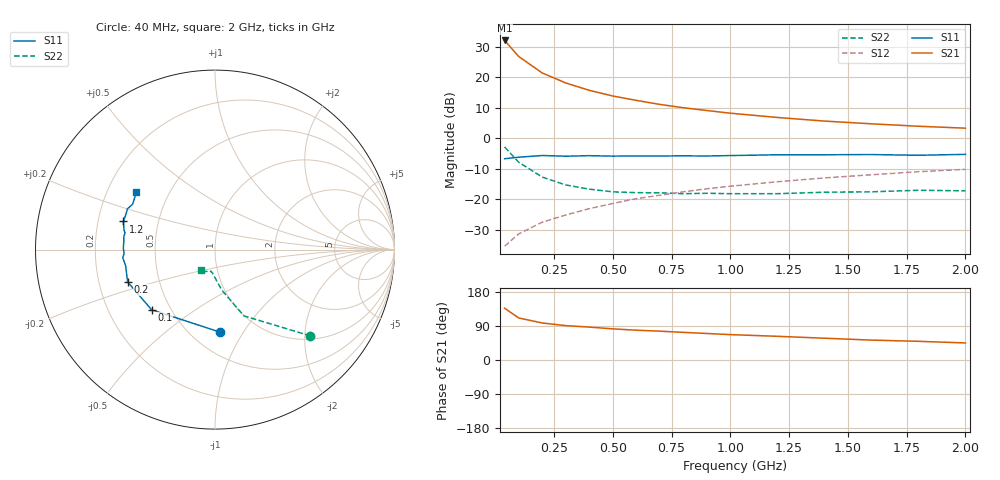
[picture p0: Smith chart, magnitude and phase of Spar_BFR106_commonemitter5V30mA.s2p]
! Filename:  BFR106B.S2P  Version:  2.0
! NXP part #: BFR106  Date: Jun 1990
! Bias condition: Vce=5V, Ic=30mA
#  MHz  S  MA  R  50
! Freq  S11  S21  S12  S22  !GUM [dB]
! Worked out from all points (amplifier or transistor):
!   16 points, 40 MHz to 2 GHz, reference 50 ohm
!   highest |S21| = 32.0 dB at 40 MHz (marker M1)
!   |S21| within 3 dB of that: start of sweep to 74.27 MHz
!   unconditionally stable (mu >= 1): 328 MHz to 1.938 GHz
!   at 200 MHz: K = 0.86, MSG = 24.4 dB, |S12| = -27.5 dB
!   at 800 MHz: K = 1.06, MAG = 12.2 dB, |S12| = -17.6 dB
!   at 2 GHz: K = 0.99, MSG = 6.7 dB, |S12| = -10.2 dB
!   S11 on the Smith chart (normalised r, x): 40 MHz: 0.68, -0.79; 100 MHz: 0.39, -0.34; 200 MHz: 0.33, -0.16; 1.2 GHz: 0.31, +0.14; 2 GHz: 0.33, +0.29
40  0.46 -86.7  39.78 136.7  0.017 63.4  0.717 -42.1
100  0.487 -136.5  21.73 110.9  0.027 56.5  0.403 -66.4
200  0.519 -159.7  11.68 97.7  0.042 63.0  0.23 -80.3
300  0.506 -169.8  8.005 90.7  0.055 66.6  0.171 -87.5
400  0.516 -175.0  6.068 86.8  0.07 69.2  0.146 -92.3
500  0.507 -177.4  4.899 82.2  0.085 70.6  0.132 -95.7
600  0.511 179.1  4.153 78.6  0.102 70.9  0.128 -97.9
700  0.51 175.4  3.568 76.1  0.116 71.1  0.127 -98.9
800  0.513 171.6  3.146 72.9  0.132 71.2  0.123 -100.1
900  0.51 169.3  2.834 70.0  0.148 71.2  0.125 -99.7
1000  0.518 168.1  2.561 67.0  0.163 70.2  0.123 -101.6
1200  0.534 162.9  2.18 62.5  0.193 69.3  0.123 -106.2
1400  0.534 158.3  1.902 57.5  0.223 67.6  0.13 -110.6
1600  0.538 155.0  1.716 52.5  0.251 66.5  0.132 -113.0
1800  0.524 151.1  1.565 49.3  0.282 64.7  0.14 -117.5
2000  0.542 144.0  1.456 45.0  0.308 63.2  0.137 -123.5
